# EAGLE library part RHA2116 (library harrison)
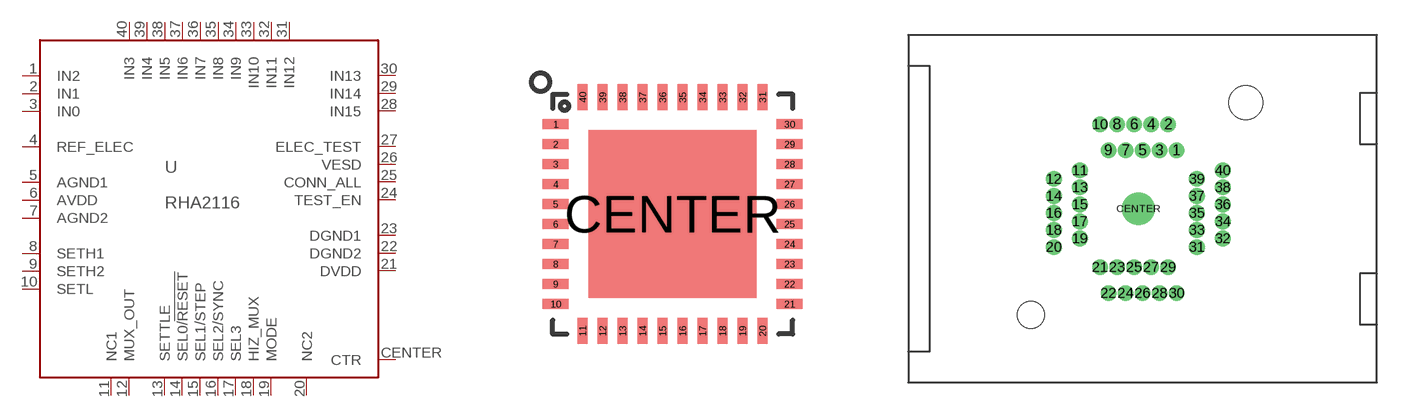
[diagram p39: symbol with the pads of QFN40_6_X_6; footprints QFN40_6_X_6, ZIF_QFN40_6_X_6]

Designator prefix U

## RHA2116QFN  [QFN40_6_X_6]
1  IN2  in
2  IN1  in
3  IN0  in
4  REF_ELEC  in
5  AGND1  pwr
6  AVDD  pwr
7  AGND2  pwr
8  SETH1  pas
9  SETH2  pas
10  SETL  pas
11  NC1  nc
12  MUX_OUT  hiz
13  SETTLE  in
14  SEL0/!RESET!  in
15  SEL1/STEP  in
16  SEL2/SYNC
17  SEL3
18  HIZ_MUX  in
19  MODE  in
20  NC2  nc
21  DVDD  pwr
22  DGND2  pwr
23  DGND1  pwr
24  TEST_EN  in
25  CONN_ALL  in
26  VESD  pwr
27  ELEC_TEST  in
28  IN15  in
29  IN14  in
30  IN13  in
31  IN12  in
32  IN11  in
33  IN10  in
34  IN9  in
35  IN8  in
36  IN7  in
37  IN6  in
38  IN5  in
39  IN4  in
40  IN3  in
CENTER  CTR  pwr

## RHA2116ZIF  [ZIF_QFN40_6_X_6]
Pads as for QFN40_6_X_6

## Footprint QFN40_6_X_6 (pad centres in mm)
smd 0.65 x 0.25: 1 -2.925,2.25; 2 -2.925,1.75; 3 -2.925,1.25; 4 -2.925,0.75; 5 -2.925,0.25; 6 -2.925,-0.25; 7 -2.925,-0.75; 8 -2.925,-1.25; 9 -2.925,-1.75; 10 -2.925,-2.25; 21 2.925,-2.25; 22 2.925,-1.75; 23 2.925,-1.25; 24 2.925,-0.75; 25 2.925,-0.25; 26 2.925,0.25; 27 2.925,0.75; 28 2.925,1.25; 29 2.925,1.75; 30 2.925,2.25
smd 0.25 x 0.65: 11 -2.25,-2.925; 12 -1.75,-2.925; 13 -1.25,-2.925; 14 -0.75,-2.925; 15 -0.25,-2.925; 16 0.25,-2.925; 17 0.75,-2.925; 18 1.25,-2.925; 19 1.75,-2.925; 20 2.25,-2.925; 31 2.25,2.925; 32 1.75,2.925; 33 1.25,2.925; 34 0.75,2.925; 35 0.25,2.925; 36 -0.25,2.925; 37 -0.75,2.925; 38 -1.25,2.925; 39 -1.75,2.925; 40 -2.25,2.925
smd 4.2 x 4.2: CENTER 0,0

## Footprint ZIF_QFN40_6_X_6 (pad centres in mm)
drill 0.41 pad 0.813: 1 2.25,3.43; 2 1.75,4.955; 3 1.25,3.43; 4 0.75,4.955; 5 0.25,3.43; 6 -0.25,4.955; 7 -0.75,3.43; 8 -1.25,4.955; 9 -1.75,3.43; 10 -2.25,4.955; 11 -3.43,2.25; 12 -4.955,1.75; 13 -3.43,1.25; 14 -4.955,0.75; 15 -3.43,0.25; 16 -4.955,-0.25; 17 -3.43,-0.75; 18 -4.955,-1.25; 19 -3.43,-1.75; 20 -4.955,-2.25; 21 -2.25,-3.43; 22 -1.75,-4.955; 23 -1.25,-3.43; 24 -0.75,-4.955; 25 -0.25,-3.43; 26 0.25,-4.955; 27 0.75,-3.43; 28 1.25,-4.955; 29 1.75,-3.43; 30 2.25,-4.955; 31 3.43,-2.25; 32 4.955,-1.75; 33 3.43,-1.25; 34 4.955,-0.75; 35 3.43,-0.25; 36 4.955,0.25; 37 3.43,0.75; 38 4.955,1.25; 39 3.43,1.75; 40 4.955,2.25
drill 1.02 pad 1.93: CENTER 0,0
hole 1.6 at -6.31,-6.23
hole 2 at 6.31,6.23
